[IBIS VER]   5.0
[File Name]   f28p551pz.ibs
[File Rev]   1.0
[Date]   August 04, 2025
[Source]   File originated at Texas Instruments
[Copyright]   (c) 2012, Texas Instruments Inc.
[Component]   f28p551pz
[Manufacturer]  Texas Instruments
[Package]
| Variable   Typ   Min   Max
R_pkg  2.90E-01  1.21E-01  3.50E-01
L_pkg  6.67E-09  4.61E-09  8.17E-09
C_pkg  9.64E-15  7.65E-15  1.20E-14
[Pin]   signal_name   model_name   R_pin   L_pin   C_pin
   1   A16,B16,C16,GPIO28   BCF3385DSHYPBFZ_LC  3.44E-01  8.11E-09  1.11E-14
   2   XRSn   BQ0491FS_USF  3.28E-01  7.84E-09  1.07E-14
   3   VDDIO   NC  3.22E-01  7.67E-09  1.05E-14
   4   VDD   NC  1.73E-01  6.02E-09  9.16E-15
   5   VSS   NC  1.70E-01  5.88E-09  8.93E-15
   6   GPIO47   BCF3385DSHYPBFZ_LC_USF  2.96E-01  7.07E-09  9.69E-15
   7   GPIO48   BCF3385DSHYPBFZ_LC_USF  2.93E-01  6.94E-09  9.47E-15
   8   GPIO49   BCF3385DSHYPBFZ_LC_USF  2.86E-01  6.76E-09  9.21E-15
   9   GPIO50   BCF3385DSHYPBFZ_LC_USF  2.81E-01  6.60E-09  8.97E-15
   10   GPIO51   BCF3385DSHYPBFZ_LC_USF  2.78E-01  6.45E-09  8.75E-15
   11   GPIO52   BCF3385DSHYPBFZ_LC_USF  2.76E-01  6.33E-09  8.53E-15
   12   GPIO53   BCF3385DSHYPBFZ_LC_USF  2.76E-01  6.22E-09  8.33E-15
   13   GPIO54   BCF3385DSHYPBFZ_LC_USF  2.78E-01  6.12E-09  9.69E-15
   14   A6,D14,E14,GPIO228   BCF3385DSHYPBFZ_LC_USF  2.81E-01  6.26E-09  8.37E-15
   15   B2,C6,E12,GPIO226   BCF3385DSHYPBFZ_LC_USF  2.85E-01  6.42E-09  8.60E-15
   16   B3,GPIO242,PGA2_INP   BCF3385DSHYPBFZ_LC_USF  2.91E-01  6.59E-09  8.85E-15
   17   A2,B6,C9,GPIO224,PGA1_INP   BCF3385DSHYPBFZ_LC  2.91E-01  6.70E-09  9.05E-15
   18   A3,B9,C7,PGA1_INM   ICF33SHYPB_LC  2.86E-01  6.75E-09  9.21E-15
   19   A14,B14,C4,PGA1_OUT   ICF33SHYPB_LC  2.84E-01  6.84E-09  9.39E-15
   20   A11,B10,C0,PGA2_OUT   ICF33SHYPB_LC  2.90E-01  7.01E-09  9.64E-15
   21   B12,C2,PGA2_INM   ICF33SHYPB_LC  2.96E-01  7.18E-09  9.89E-15
   22   A1,B7,D11,DACB_OUT   ICF33SHYPB_LC  3.05E-01  7.39E-09  1.02E-14
   23   A0,B15,C15,DACA_OUT   ICF33SHYPB_LC  3.17E-01  7.62E-09  1.05E-14
   24   D20,E20,VREFHI   ICF33SHYPB_LC  3.27E-01  7.83E-09  1.07E-14
   25   D20,E20,VREFHI   ICF33SHYPB_LC  1.88E-01  6.50E-09  9.87E-15
   26   A13,B13,C13,D13,E13,VREFLO   ICF33SHYPB_LC  1.90E-01  6.57E-09  9.98E-15
   27   A13,B13,C13,D13,E13,VREFLO   ICF33SHYPB_LC  3.35E-01  7.95E-09  1.09E-14
   28   A12,C5   ICF33SHYPB_LC  3.24E-01  7.73E-09  1.06E-14
   29   C1,E11,PGA3_INP   ICF33SHYPB_LC  3.17E-01  7.55E-09  1.03E-14
   30   B11,D16,E16,PGA3_INM   ICF33SHYPB_LC  3.18E-01  7.45E-09  1.01E-14
   31   A7,B30,C3,D12,E30   ICF33SHYPB_LC  3.07E-01  7.22E-09  9.85E-15
   32   B5,D15,E15,PGA3_OUT   ICF33SHYPB_LC  3.11E-01  7.16E-09  9.68E-15
   33   VSSA   NC  1.21E-01  5.09E-09  8.03E-15
   34   VDDA   NC  1.21E-01  4.98E-09  7.82E-15
   35   A5   ICF33SHYPB_LC  3.03E-01  6.75E-09  9.01E-15
   36   A4,B8   ICF33SHYPB_LC  3.02E-01  6.62E-09  8.79E-15
   37   A8   ICF33SHYPB_LC  3.01E-01  6.51E-09  8.59E-15
   38   A9,GPIO227   BCF3385DSHYPBFZ_LC  3.04E-01  6.43E-09  9.97E-15
   39   B4,C8,GPIO236   BCF3385DSHYPBFZ_LC  3.00E-01  6.28E-09  9.68E-15
   40   A10,B1,C10,GPIO230   BCF3385DSHYPBFZ_LC  2.98E-01  6.14E-09  9.41E-15
   41   B0,C11,GPIO253   BCF3385DSHYPBFZ_LC  2.97E-01  6.02E-09  9.15E-15
   42   C14,GPIO247   BCF3385DSHYPBFZ_LC  2.98E-01  5.92E-09  8.90E-15
   43   GPIO55   BCF3385DSHYPBFZ_LC  3.00E-01  5.84E-09  8.66E-15
   44   GPIO60   BCF3385DSHYPBFZ_LC  3.04E-01  5.77E-09  8.44E-15
   45   VSS   NC  1.67E-01  4.61E-09  1.10E-14
   46   GPIO62   BCF3385DSHYPBFZ_LC  2.99E-01  5.84E-09  1.16E-14
   47   GPIO63   BCF3385DSHYPBFZ_LC  3.05E-01  5.78E-09  1.12E-14
   48   A17,B17,C17,CMP1_DACL,GPIO20   BCF3385DSHYPBFZ_LC  3.13E-01  5.73E-09  1.09E-14
   49   A18,B18,C18,GPIO21   BCF3385DSHYPBFZ_LC  3.23E-01  5.71E-09  1.05E-14
   50   A19,B19,C19,GPIO13   BCF3385DSHYPBFZ_LC  3.35E-01  5.85E-09  1.02E-14
   51   A20,B20,C20,GPIO12   BCF3385DSHYPBFZ_LC  3.50E-01  8.17E-09  1.11E-14
   52   A24,D0,E0,GPIO11   BCF3385DSHYPBFZ_LC  3.21E-01  7.77E-09  1.07E-14
   53   B24,D1,E1,GPIO33   BCF3385DSHYPBFZ_LC  3.06E-01  7.50E-09  1.04E-14
   54   C24,D2,E2,GPIO16   BCF3385DSHYPBFZ_LC  2.96E-01  7.29E-09  1.01E-14
   55   A25,D3,E3,GPIO17   BCF3385DSHYPBFZ_LC  2.89E-01  7.11E-09  9.84E-15
   56   B25,D4,E4,GPIO24   BCF3385DSHYPBFZ_LC  2.84E-01  6.95E-09  9.60E-15
   57   GPIO25   BCF3385DSHYPBFZ_LC  2.82E-01  6.82E-09  9.38E-15
   58   GPIO26   BCF3385DSHYPBFZ_LC  2.81E-01  6.70E-09  9.17E-15
   59   GPIO27   BCF3385DSHYPBFZ_LC  2.81E-01  6.59E-09  8.97E-15
   60   TCK   BCF3355DSHYPBFZ_TMS_USF  2.81E-01  6.49E-09  8.77E-15
   61   GPIO37/TDO   BCPF335585DSHYPBFZ  2.83E-01  6.39E-09  8.58E-15
   62   TMS   BCF3355DSHYPBFZ_TMS  2.86E-01  6.32E-09  8.41E-15
   63   GPIO35/TDI   BCF3385DSHYPBFZ_LC  2.91E-01  6.25E-09  9.79E-15
   64   GPIO32   BQ3320HYPBFZ_3VSBLK_5FS_LC  2.94E-01  6.40E-09  8.47E-15
   65   GPIO56   BCF3385DSHYPBFZ_LC  2.96E-01  6.53E-09  8.69E-15
   66   GPIO57   BCF3385DSHYPBFZ_LC  3.04E-01  6.72E-09  8.94E-15
   67   GPIO58   BCF3385DSHYPBFZ_LC  3.13E-01  6.92E-09  9.21E-15
   68   GPIO18,X2   BCF3385DSHYPBFZ_LC  3.18E-01  7.08E-09  9.46E-15
   69   GPIO19,X1   BCPF335585DSHYPBFZ  3.07E-01  7.07E-09  9.57E-15
   70   VDDIO   NC  3.19E-01  7.31E-09  9.86E-15
   71   VDD   NC  1.73E-01  5.92E-09  8.96E-15
   72   VSS   NC  1.30E-01  5.58E-09  8.83E-15
   73   VREGENZ   IQ0440FS_VREGENZ_USF  3.21E-01  7.66E-09  1.05E-14
   74   GPIO8   BCF3385DSHYPBFZ_LC  3.31E-01  7.87E-09  1.08E-14
   75   GPIO4   BCF3385DSHYPBFZ_LC  3.39E-01  8.06E-09  1.10E-14
   76   GPIO3  BQ3320HYPBFZ_3VSBLK_5FS_LC  3.45E-01  8.17E-09  1.12E-14
   77   GPIO2  BQ3320HYPBFZ_3VSBLK_5FS_LC  3.42E-01  8.03E-09  1.09E-14
   78   GPIO1   BCF3385DSHYPBFZ_LC  3.36E-01  7.86E-09  1.07E-14
   79   GPIO0   BCF3385DSHYPBFZ_LC  3.26E-01  7.64E-09  1.04E-14
   80   GPIO40   BCF3385DSHYPBFZ_LC  3.17E-01  7.44E-09  1.01E-14
   81   GPIO23   BCF3385DSHYPBFZ_LC  3.13E-01  7.29E-09  9.90E-15
   82   GPIO41   BCF3385DSHYPBFZ_LC  3.09E-01  7.13E-09  9.66E-15
   83   GPIO22   BCF3385DSHYPBFZ_LC  3.06E-01  7.00E-09  9.44E-15
   84   GPIO7   BCF3385DSHYPBFZ_LC  3.03E-01  6.85E-09  9.21E-15
   85   GPIO44   BCF3385DSHYPBFZ_LC  3.07E-01  6.79E-09  9.04E-15
   86   VSS   NC  1.69E-01  5.25E-09  7.78E-15
   87   VDD   NC  1.78E-01  5.23E-09  7.65E-15
   88   VDDIO   NC  3.18E-01  6.57E-09  1.01E-14
   89   GPIO5   BCF3385DSHYPBFZ_LC  3.09E-01  6.37E-09  9.75E-15
   90   GPIO9  BQ3320HYPBFZ_3VSBLK_5FS_LC  3.03E-01  6.20E-09  9.45E-15
   91   GPIO61   BCF3385DSHYPBFZ_LC_USF  3.02E-01  6.07E-09  9.19E-15
   92   GPIO59   BCF3385DSHYPBFZ_LC_USF  2.97E-01  5.91E-09  8.89E-15
   93   GPIO10   BCF3385DSHYPBFZ_LC_USF  2.93E-01  5.77E-09  8.61E-15
   94   GPIO34   BCF3385DSHYPBFZ_LC_USF  2.91E-01  5.64E-09  8.34E-15
   95   GPIO15   BCF3385DSHYPBFZ_LC_USF  2.91E-01  5.89E-09  1.20E-14
   96   GPIO14   BCF3385DSHYPBFZ_LC_USF  2.92E-01  5.77E-09  1.16E-14
   97   GPIO6   BCF3385DSHYPBFZ_LC_USF  2.95E-01  5.68E-09  1.12E-14
   98   GPIO30   BCF3385DSHYPBFZ_LC  3.01E-01  5.61E-09  1.08E-14
   99   GPIO31   BCF3385DSHYPBFZ_LC  3.14E-01  5.62E-09  1.05E-14
   100   GPIO29   BCF3385DSHYPBFZ_LC  3.28E-01  5.78E-09  1.01E-14
| End of package information
|   Component BQ0491FS_USF
[Component]   BQ0491FS_USF
[Manufacturer]   Texas Instruments
[Package]
|  variable   typ   min   max
R_pkg   0   0   0
L_pkg   0   0   0
C_pkg   0   0   0
[Pin]   signal_name   model_name   R_pin   L_pin   C_pin
VSS   VSS   GND
VDDS   VDDS   POWER
PAD   PAD   BQ0491FS_USF
[Model Selector] BQ0491FS_USF
WK_PU_ON_WITH_RX_3P3  Cell operated at 3.3(nom)
|WK_PU_ON_WITH_RX_3P3; WEAK_PULLUP_ON_WITH_RX
OPEN_DRAIN_MODE_3P3  Cell operated at 3.3(nom)
|   Component BCPF335585DSHYPBFZ
[Component]   BCPF335585DSHYPBFZ
[Manufacturer]   Texas Instruments
[Package]
|  variable   typ   min   max
R_pkg   0   0   0
L_pkg   0   0   0
C_pkg   0   0   0
[Pin]   signal_name   model_name   R_pin   L_pin   C_pin
VSS   VSS   GND
VDDS   VDDS   POWER
PAD   PAD   BCPF335585DSHYPBFZ
[Model Selector] BCPF335585DSHYPBFZ
BCPF_WK_PU_ON_3P3  Cell operated at 3.3(nom)
|BCPF_WK_PU_ON_3P3; WEAK_PULLUP_ON
BCPF_DRIVER_MODE_4MA_3P3  Cell operated at 3.3(nom)
|BCPF_DRIVER_MODE_4MA_3P3
BCPF_DRIVER_MODE_2MA_3P3  Cell operated at 3.3(nom)
|BCPF_DRIVER_MODE_2MA_3P3
BCPF_WK_PD_ON_3P3  Cell operated at 3.3(nom)
|   Component ICF33SHYPB_LC
[Component]   ICF33SHYPB_LC
[Manufacturer]   Texas Instruments
[Package]
|  variable   typ   min   max
R_pkg   0   0   0
L_pkg   0   0   0
C_pkg   0   0   0
[Pin]   signal_name   model_name   R_pin   L_pin   C_pin
VSS   VSS   GND
VDDS   VDDS   POWER
PAD   PAD   ICF33SHYPB_LC
[Model Selector] ICF33SHYPB_LC
ICF_RECEIVER_MODE_3P3  Cell operated at 3.3(nom)
|ICF_RECEIVER_MODE_3P3; RECEIVER_MODE
ICF_WK_PU_ON_3P3  Cell operated at 3.3(nom)
|ICF_WK_PU_ON_3P3; WEAK_PULLUP_ON
ICF_WK_PD_ON_3P3  Cell operated at 3.3(nom)
|   Component BCF3385DSHYPBFZ_LC_USF
[Component]   BCF3385DSHYPBFZ_LC_USF
[Manufacturer]   Texas Instruments
[Package]
|  variable   typ   min   max
R_pkg   0   0   0
L_pkg   0   0   0
C_pkg   0   0   0
[Pin]   signal_name   model_name   R_pin   L_pin   C_pin
VSS   VSS   GND
VDDS   VDDS   POWER
PAD   PAD   BCF3385DSHYPBFZ_LC_USF
[Model Selector] BCF3385DSHYPBFZ_LC_USF
BCF_WK_PU_ON_3P3  Cell operated at 3.3(nom)
|BCF_WK_PU_ON_3P3; WEAK_PULLUP_ON
BCF_WK_PD_ON_3P3  Cell operated at 3.3(nom)
|BCF_WK_PD_ON_3P3; WEAK_PULLDOWN_ON
BCF_DRIVER_MODE_3P3  Cell operated at 3.3(nom)
|BCF_DRIVER_MODE_3P3
BCF_RECEIVER_MODE_3P3  Cell operated at 3.3(nom)
|   Component BCF3355DSHYPBFZ_TMS_USF
[Component]   BCF3355DSHYPBFZ_TMS_USF
[Manufacturer]   Texas Instruments
[Package]
|  variable   typ   min   max
R_pkg   0   0   0
L_pkg   0   0   0
C_pkg   0   0   0
[Pin]   signal_name   model_name   R_pin   L_pin   C_pin
VSS   VSS   GND
VDDS   VDDS   POWER
PAD   PAD   BCF3355DSHYPBFZ_TMS_USF
[Model Selector] BCF3355DSHYPBFZ_TMS_USF
TMS_WK_PU_ON_3P3  Cell operated at 3.3(nom)
|TMS_WK_PU_ON_3P3; WEAK_PULLUP_ON
TMS_DRIVER_3P3  Cell operated at 3.3(nom)
|TMS_DRIVER_3P3
TMS_WK_PD_ON_3P3  Cell operated at 3.3(nom)
|   Component BCF3385DSHYPBFZ_LC
[Component]   BCF3385DSHYPBFZ_LC
[Manufacturer]   Texas Instruments
[Package]
|  variable   typ   min   max
R_pkg   0   0   0
L_pkg   0   0   0
C_pkg   0   0   0
[Pin]   signal_name   model_name   R_pin   L_pin   C_pin
VSS   VSS   GND
VDDS   VDDS   POWER
PAD   PAD   BCF3385DSHYPBFZ_LC
[Model Selector] BCF3385DSHYPBFZ_LC
BCF_WK_PU_ON_3P3  Cell operated at 3.3(nom)
|BCF_WK_PU_ON_3P3; WEAK_PULLUP_ON
BCF_WK_PD_ON_3P3  Cell operated at 3.3(nom)
|BCF_WK_PD_ON_3P3; WEAK_PULLDOWN_ON
BCF_DRIVER_MODE_3P3  Cell operated at 3.3(nom)
|BCF_DRIVER_MODE_3P3
BCF_RECEIVER_MODE_3P3  Cell operated at 3.3(nom)
|BCF_RECEIVER_MODE_3P3; RECEIVER_MODE
|   Component IQ0440FS_VREGENZ_USF
[Component]   IQ0440FS_VREGENZ_USF
[Manufacturer]   Texas Instruments
[Package]
|  variable   typ   min   max
R_pkg   0   0   0
L_pkg   0   0   0
C_pkg   0   0   0
[Pin]   signal_name   model_name   R_pin   L_pin   C_pin
VSS   VSS   GND
VDDS   VDDS   POWER
PAD   PAD   IQ0440FS_VREGENZ_USF
[Model Selector] IQ0440FS_VREGENZ_USF
VREGENZ_WK_PD_ON_3P3  Cell operated at 3.3(nom)
|VREGENZ_WK_PD_ON_3P3; WEAK_PULLDOWN_ON
VREGENZ_WK_PD_OFF_3P3  Cell operated at 3.3(nom)
|   Component BCF3355DSHYPBFZ_TMS
[Component]   BCF3355DSHYPBFZ_TMS
[Manufacturer]   Texas Instruments
[Package]
|  variable   typ   min   max
R_pkg   0   0   0
L_pkg   0   0   0
C_pkg   0   0   0
[Pin]   signal_name   model_name   R_pin   L_pin   C_pin
VSS   VSS   GND
VDDS   VDDS   POWER
PAD   PAD   BCF3355DSHYPBFZ_TMS
[Model Selector] BCF3355DSHYPBFZ_TMS
TMS_WK_PU_ON_3P3  Cell operated at 3.3(nom)
|TMS_WK_PU_ON_3P3; WEAK_PULLUP_ON
TMS_DRIVER_3P3  Cell operated at 3.3(nom)
|TMS_DRIVER_3P3
TMS_WK_PD_ON_3P3  Cell operated at 3.3(nom)
|TMS_WK_PD_ON_3P3; WEAK_PULLDOWN_ON
|   Component BQ3320HYPBFZ_3VSBLK_5FS_LC
[Component] BQ3320HYPBFZ_3VSBLK_5FS_LC
[Manufacturer] Texas Instruments
[Package]
| variable   typ   min   max
R_pkg   0.0   0.0   0.0
L_pkg   0.0H   0.0H   0.0H
C_pkg   0.0F   0.0F   0.0F
[Pin]  signal_name   model_name   R_pin   L_pin   C_pin
PAD   PAD   BQ3320HYPBFZ_3VSBLK_5FS_LC
VDDS   VDDS   Power
VSS   VSS   Gnd
A   A   NC
GZ   GZ   NC
[Model Selector] BQ3320HYPBFZ_3VSBLK_5FS_LC
BQ3320HYPBFZ_3VSBLK_5FS_LC_M0_D0 I/O model with Mode = 0 and Drive = 0
BQ3320HYPBFZ_3VSBLK_5FS_LC_M0_D1 I/O model with Mode = 0 and Drive = 1
BQ3320HYPBFZ_3VSBLK_5FS_LC_M1_D0 I/O model with Mode = 1 and Drive = 0
BQ3320HYPBFZ_3VSBLK_5FS_LC_M1_D1 I/O model with Mode = 1 and Drive = 1
BQ3320HYPBFZ_3VSBLK_5FS_LC_PDON I/O model with Pulldown on PI=0 PSEL=0
BQ3320HYPBFZ_3VSBLK_5FS_LC_PUON I/O model with Pullup on PI=0 PSEL=0
| Models and submodels in the file (24): WK_PU_ON_WITH_RX_3P3 (Input), OPEN_DRAIN_MODE_3P3 (I/O_open_drain), BCPF_WK_PU_ON_3P3 (Input), BCPF_DRIVER_MODE_4MA_3P3 (I/O), BCPF_DRIVER_MODE_2MA_3P3 (I/O), BCPF_WK_PD_ON_3P3 (Input), ICF_RECEIVER_MODE_3P3 (Input), ICF_WK_PU_ON_3P3 (Input), ICF_WK_PD_ON_3P3 (Input), BCF_WK_PU_ON_3P3 (Input), BCF_WK_PD_ON_3P3 (Input), BCF_DRIVER_MODE_3P3 (I/O), BCF_RECEIVER_MODE_3P3 (Input), TMS_WK_PU_ON_3P3 (Input), TMS_DRIVER_3P3 (I/O), TMS_WK_PD_ON_3P3 (Input), VREGENZ_WK_PD_ON_3P3 (Input), VREGENZ_WK_PD_OFF_3P3 (Input), BQ3320HYPBFZ_3VSBLK_5FS_LC_M0_D0 (I/O), BQ3320HYPBFZ_3VSBLK_5FS_LC_M0_D1 (I/O), BQ3320HYPBFZ_3VSBLK_5FS_LC_M1_D0 (I/O), BQ3320HYPBFZ_3VSBLK_5FS_LC_M1_D1 (I/O), BQ3320HYPBFZ_3VSBLK_5FS_LC_PDON (Input), BQ3320HYPBFZ_3VSBLK_5FS_LC_PUON (Input)
